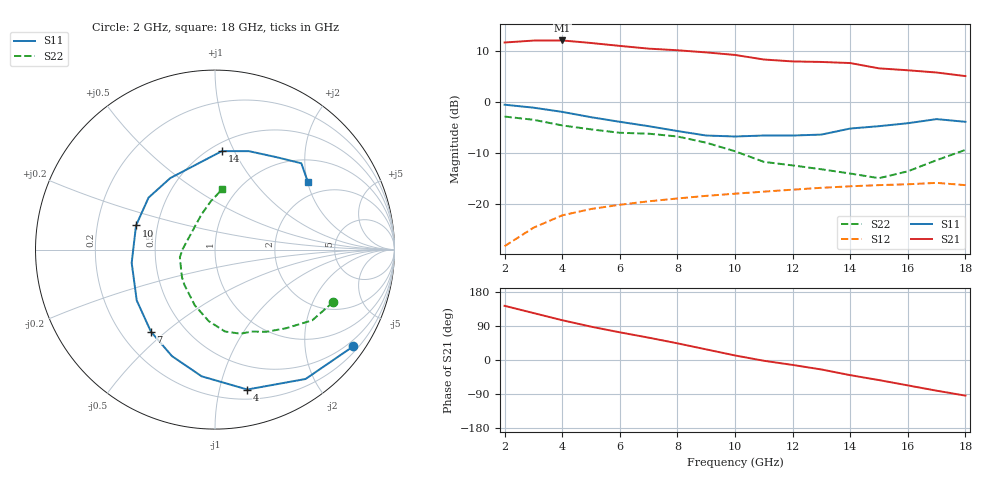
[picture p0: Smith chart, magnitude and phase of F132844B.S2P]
!ATF-13284
!S-PARAMETERS at Vds=4V  Id=40mA.  LAST UPDATED 07-22-92
# ghz s ma r 50
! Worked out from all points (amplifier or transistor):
!   17 points, 2 GHz to 18 GHz, reference 50 ohm
!   highest |S21| = 12.0 dB at 4 GHz (marker M1)
!   |S21| within 3 dB of that: start of sweep to 10.19 GHz
!   unconditionally stable (mu >= 1): 9.262 GHz to 16.53 GHz; 17.66 GHz to end of sweep
!   at 4 GHz: K = 0.52, MSG = 17.1 dB, |S12| = -22.2 dB
!   at 10 GHz: K = 1.04, MAG = 12.4 dB, |S12| = -17.9 dB
!   at 18 GHz: K = 1.04, MAG = 9.4 dB, |S12| = -16.2 dB
!   S11 on the Smith chart (normalised r, x): 2 GHz: 0.34, -3.14; 4 GHz: 0.28, -1.22; 7 GHz: 0.32, -0.45; 10 GHz: 0.38, +0.13; 14 GHz: 0.57, +0.90; 18 GHz: 1.58, +2.01
2  0.94 -35.0  3.81 143.0  0.039 67.0  0.72 -24.0
3  0.88 -55.0  3.98 124.0  0.059 54.0  0.67 -36.0
4  0.8 -77.0  3.99 105.0  0.078 42.0  0.59 -48.0
5  0.71 -96.0  3.77 88.0  0.09 33.0  0.54 -58.0
6  0.64 -112.0  3.53 73.0  0.099 24.0  0.5 -66.0
7  0.58 -128.0  3.32 59.0  0.107 18.0  0.49 -73.0
8  0.52 -147.0  3.2 44.0  0.114 11.0  0.46 -83.0
9  0.47 -171.0  3.05 28.0  0.121 3.0  0.4 -95.0
10  0.46 163.0  2.88 12.0  0.127 -5.0  0.33 -110.0
11  0.47 142.0  2.6 -2.0  0.133 -10.0  0.26 -131.0
12  0.47 122.0  2.49 -13.0  0.139 -16.0  0.24 -140.0
13  0.48 105.0  2.46 -25.0  0.145 -22.0  0.22 -149.0
14  0.55 86.0  2.4 -40.0  0.15 -28.0  0.2 -168.0
15  0.58 71.0  2.13 -53.0  0.154 -36.0  0.18 179.0
16  0.62 56.0  2.04 -67.0  0.157 -43.0  0.21 111.0
17  0.68 45.0  1.94 -81.0  0.162 -52.0  0.27 95.0
18  0.64 36.0  1.79 -94.0  0.154 -69.0  0.34 83.0
